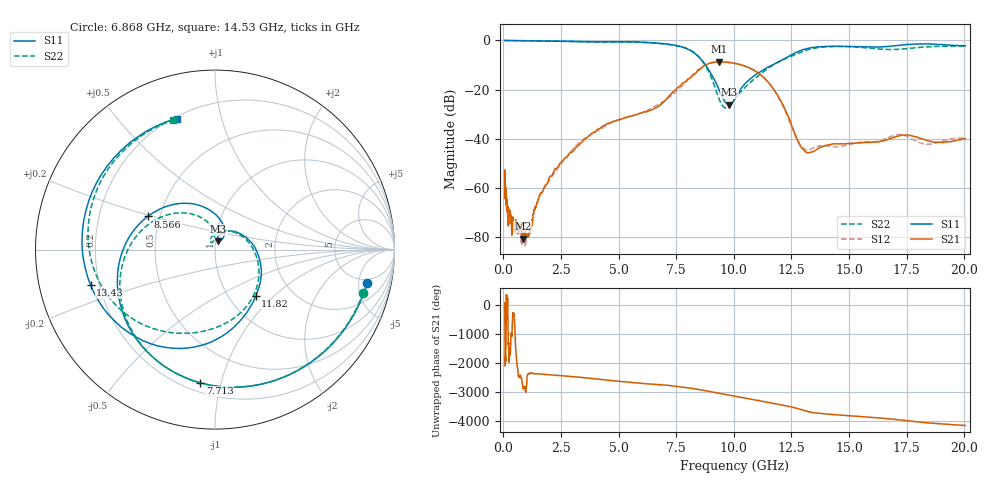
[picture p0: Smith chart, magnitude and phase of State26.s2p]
# Hz S DB R 50
!freq MagS11 AngS11 MagS21 AngS21 MagS12 AngS12 MagS22 AngS22
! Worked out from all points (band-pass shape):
!   1601 points, 50 MHz to 20.05 GHz, reference 50 ohm
!   highest |S21| = -8.65 dB at 9.372 GHz (marker M1); lowest = -80.4 dB at 836.5 MHz (marker M2)
!   |S21| within 3 dB of the highest: 8.544 GHz to 10.79 GHz (2.243 GHz wide, 23.2 % of centre)
!   lowest |S11| = -26.0 dB at 9.803 GHz (marker M3), VSWR 1.11, Z = 51.6 + j4.84 ohm
!   |S11| at or under -10 dB: 8.772 GHz to 11.66 GHz (2.884 GHz wide, 28.2 % of centre)
!   |S22| runs from -27.5 to 0.0 dB; largest |S21 - S12| = 0.019
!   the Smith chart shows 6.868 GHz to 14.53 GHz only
!   S11 on the Smith chart (normalised r, x): 6.868 GHz: 4.29, -6.45; 7.713 GHz: 0.26, -0.86; 8.566 GHz: 0.43, +0.19; 11.82 GHz: 1.32, -0.78; 13.43 GHz: 0.17, -0.14; 14.53 GHz: 0.21, +0.73
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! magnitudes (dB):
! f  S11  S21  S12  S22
! 50 MHz  0.0  -52.8  -52.2  0.0
! 73.54 MHz  0.0  -63.0  -57.9  0.0
! 78.38 MHz  0.0  -60.0  -60.3  0.0
! 135.9 MHz  0.0  -67.0  -65.1  0.0
! 217.1 MHz  0.0  -74.1  -73.0  0.0
! 293 MHz  0.0  -69.5  -72.0  0.0
! 369.6 MHz  0.0  -78.4  -76.0  0.0
! 399.9 MHz  0.0  -72.5  -74.9  -0.1
! 836.5 MHz  -0.1  -80.4  -77.9  -0.1
! 1.005 GHz  -0.1  -79.6  -80.0  -0.1
! 2.722 GHz  -0.3  -47.5  -47.3  -0.4
! 6.868 GHz  -1.2  -25.8  -25.2  -1.3
! 7.402 GHz  -1.9  -20.5  -21.5  -1.9
! 7.713 GHz  -2.5  -18.0  -18.8  -2.5
! 8.566 GHz  -7.6  -11.5  -11.1  -7.6
! 9.372 GHz  -20.4  -8.6  -8.7  -24.1
! 9.803 GHz  -26.0  -8.9  -8.9  -26.8
! 11.82 GHz  -9.2  -21.2  -21.3  -9.3
! 12.84 GHz  -4.3  -41.9  -41.8  -5.0
! 13.43 GHz  -2.8  -45.2  -43.8  -3.3
! 14.53 GHz  -2.4  -42.0  -43.2  -2.4
! 20.05 GHz  -2.2  -39.9  -39.6  -2.3
